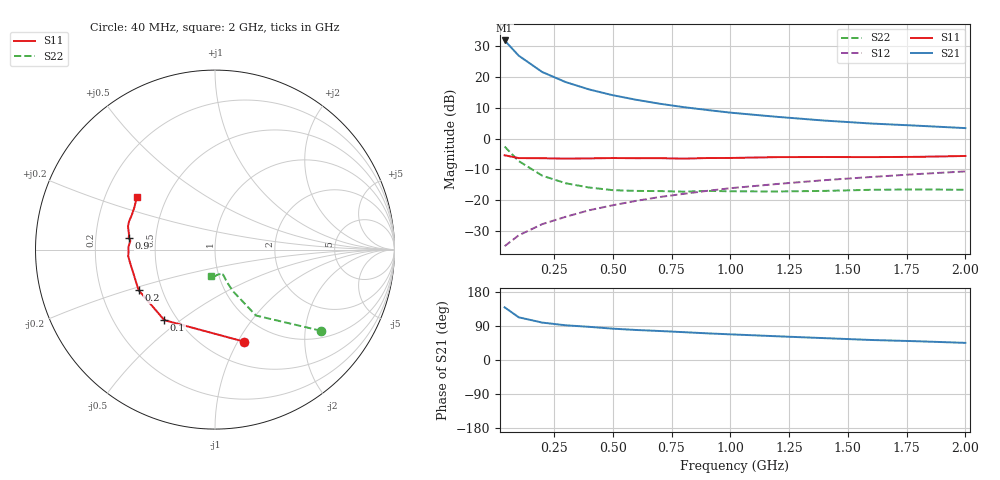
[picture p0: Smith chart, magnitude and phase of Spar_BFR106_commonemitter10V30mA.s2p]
! Filename:  BFR106F.S2P  Version:  2.0
! NXP part #: BFR106  Date: Jun 1990
! Bias condition: Vce=10V, Ic=30mA
#  MHz  S  MA  R  50
! Freq  S11  S21  S12  S22  !GUM [dB]
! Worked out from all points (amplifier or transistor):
!   16 points, 40 MHz to 2 GHz, reference 50 ohm
!   highest |S21| = 31.9 dB at 40 MHz (marker M1)
!   |S21| within 3 dB of that: start of sweep to 76.47 MHz
!   unconditionally stable (mu >= 1): 343.7 MHz to 1.942 GHz
!   at 200 MHz: K = 0.86, MSG = 24.7 dB, |S12| = -27.7 dB
!   at 800 MHz: K = 1.08, MAG = 12.4 dB, |S12| = -17.9 dB
!   at 2 GHz: K = 0.99, MSG = 7.0 dB, |S12| = -10.6 dB
!   S11 on the Smith chart (normalised r, x): 40 MHz: 0.74, -1.06; 100 MHz: 0.43, -0.44; 200 MHz: 0.37, -0.22; 900 MHz: 0.35, +0.06; 2 GHz: 0.34, +0.27
40  0.537 -72.6  39.27 139.0  0.018 64.2  0.745 -37.4
100  0.484 -125.7  22.25 112.7  0.027 57.1  0.433 -58.1
200  0.482 -152.1  12.07 98.7  0.041 61.6  0.251 -66.8
300  0.474 -165.3  8.282 91.6  0.054 64.6  0.189 -70.0
400  0.479 -171.3  6.288 87.5  0.069 67.4  0.161 -71.2
500  0.485 -175.7  5.076 82.7  0.083 69.2  0.146 -72.2
600  0.482 -178.5  4.281 79.2  0.098 70.0  0.142 -74.3
700  0.483 178.5  3.69 76.5  0.113 70.5  0.141 -74.7
800  0.474 174.0  3.257 73.5  0.127 70.4  0.138 -75.2
900  0.485 172.3  2.926 70.4  0.142 70.8  0.142 -75.6
1000  0.486 170.3  2.645 67.7  0.157 69.9  0.14 -77.2
1200  0.502 164.9  2.26 62.6  0.184 68.9  0.139 -81.1
1400  0.504 161.6  1.967 57.7  0.212 67.3  0.142 -85.9
1600  0.502 157.6  1.761 52.8  0.239 66.8  0.148 -89.2
1800  0.507 152.4  1.621 49.4  0.267 65.3  0.15 -93.7
2000  0.524 146.2  1.484 45.2  0.294 64.1  0.148 -98.9
